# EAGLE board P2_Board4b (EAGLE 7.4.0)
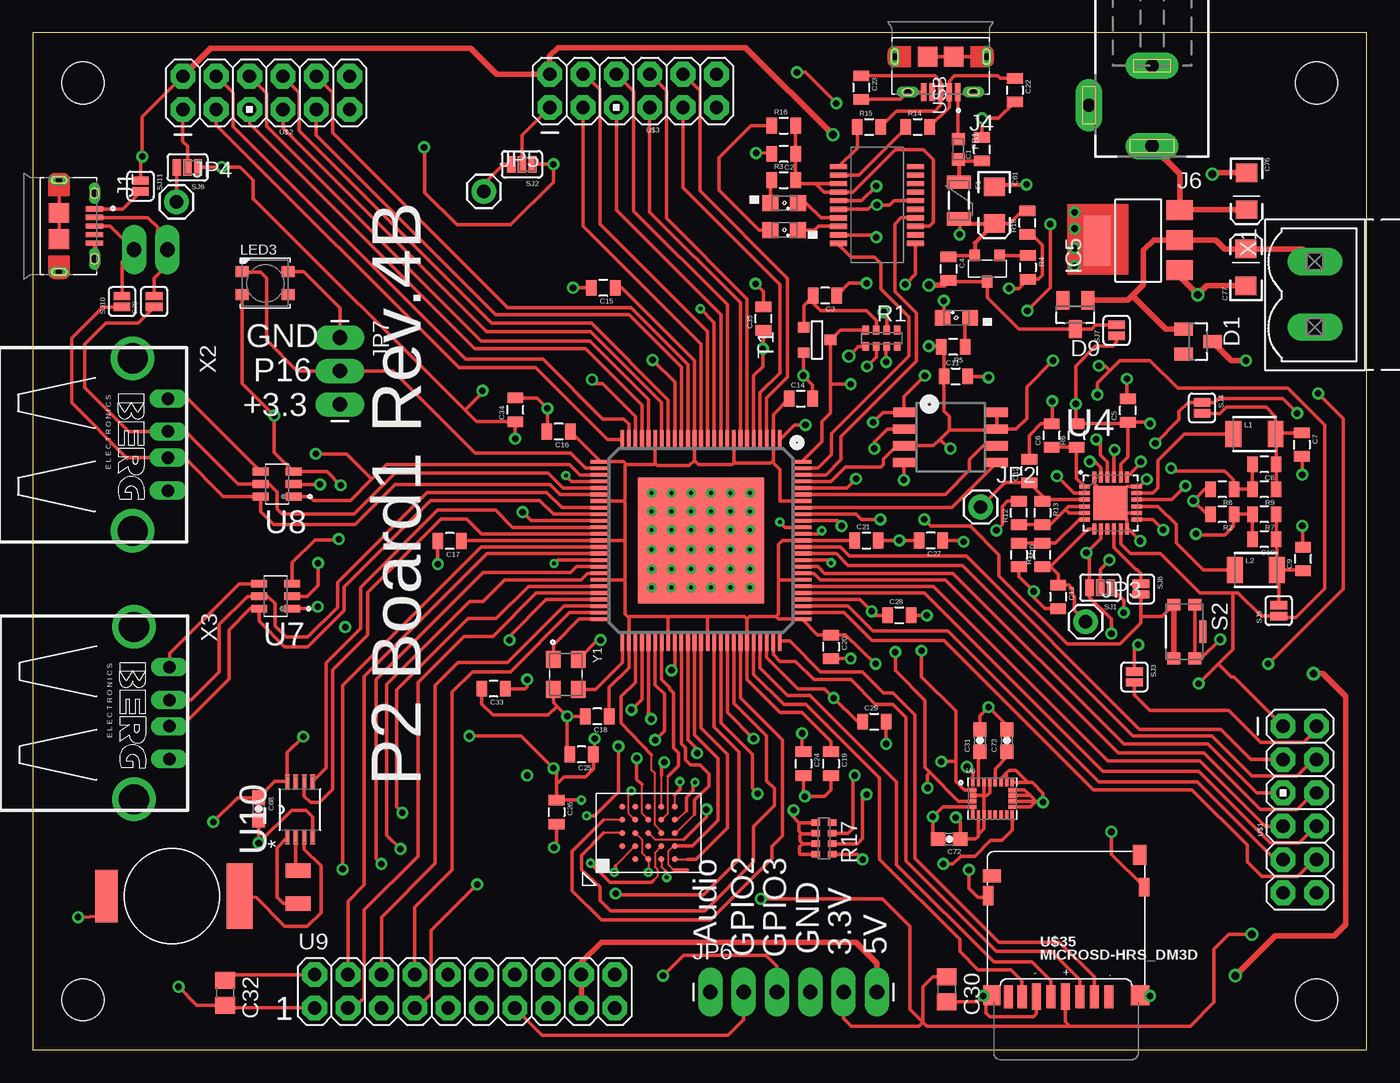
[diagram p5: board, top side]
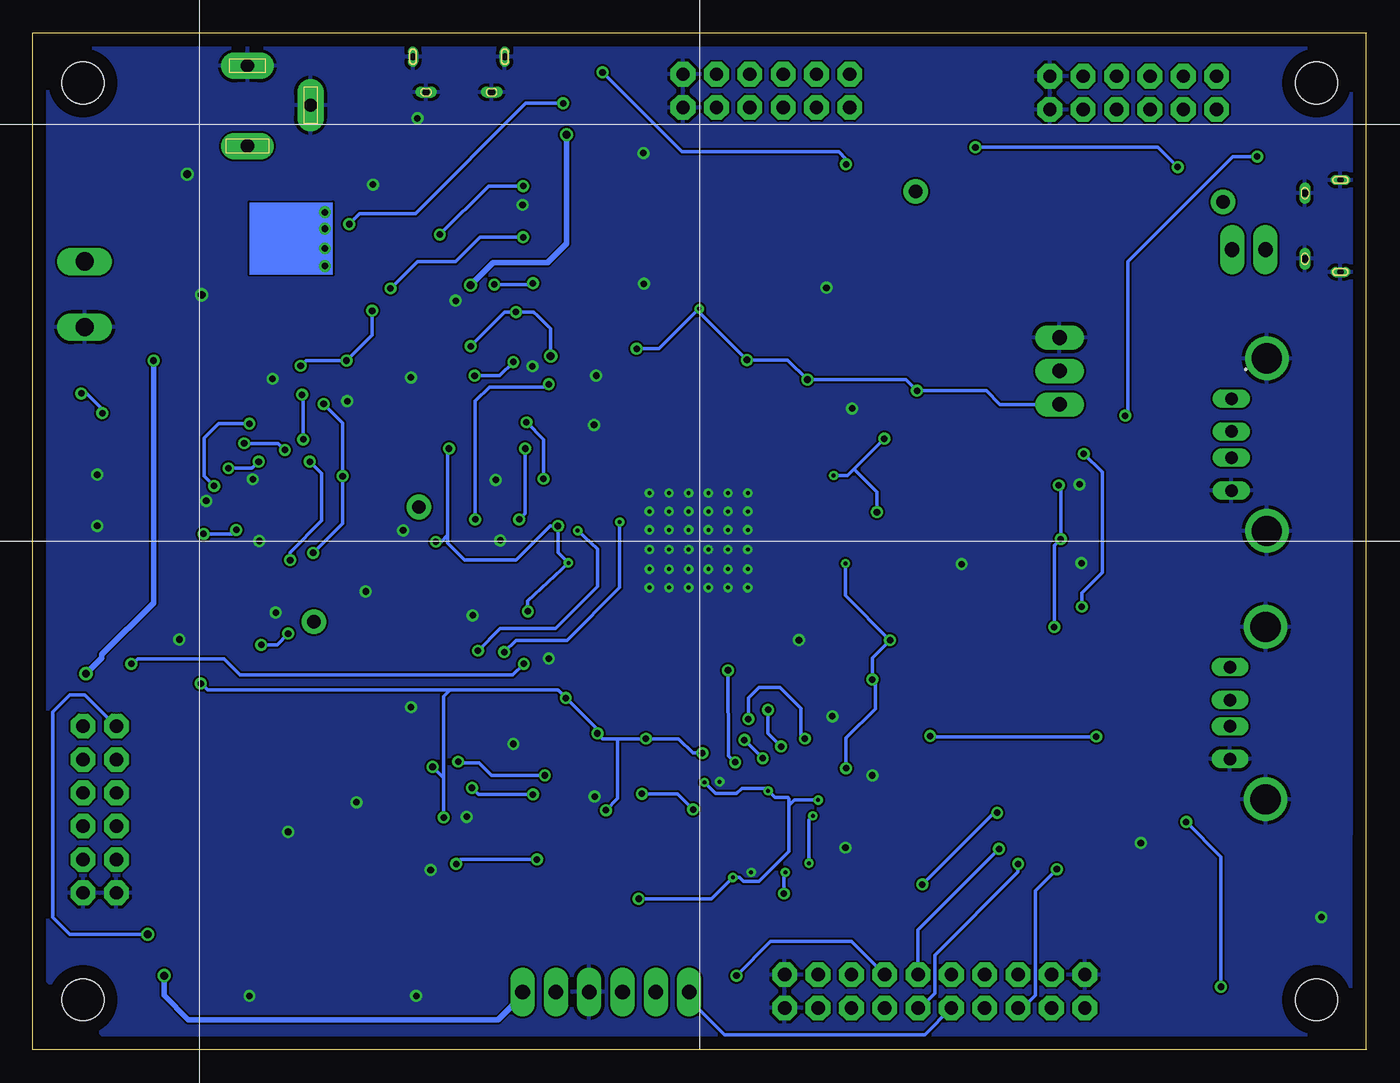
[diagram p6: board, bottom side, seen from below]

Size 101.6 x 77.47 mm. Coordinates in mm from the lower left corner, seen from the top.
Outline: 0.05,77.47 101.6,77.47 101.6,0 0.05,0
Outline: 0.05,77.47 0,77.47
Outline: 0,0 0.05,0
Outline: 0.05,0 0.05,77.47
Copper layers (1*16): Top 0.035mm / dielectric 1.5mm / Bottom 0.035mm
Design rules "default *": minimum track width 5mil, minimum drill 8mil, track to track 6mil, track to pad 6mil, pad to pad 6mil, via to via 8mil, smd to smd 8mil, copper to edge 40mil, drill to drill 8mil, minimum pad ring 4mil, minimum via ring 8mil, stop-mask expansion 4mil, vias tented up to drill 0mil, thermal gap 10mil
Net classes: 1 power: width 0.254 mm
Holes 3.2 mm at 3.81,3.81 3.81,73.66 97.79,73.66 97.79,3.81

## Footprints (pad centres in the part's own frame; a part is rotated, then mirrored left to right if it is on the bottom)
0805 = smd 0.8 x 1.2: 1 -0.9,0; 2 0.9,0
C0805 = smd 1.3 x 1.5: 1 -0.95,0; 2 0.95,0
0603-CAP = smd 1.1 x 1: 1 -0.85,0; 2 0.85,0
EIA3216 = smd 1.4 x 1.6: A 1.4,0; C -1.4,0
RAY2_SUPERCAP = smd 4 x 1.7: PNEG 0,0 | smd 5 x 2: PPOS 0,10.15
SOT23 = smd 1 x 1.4: 1 -0.95,-1.1; 2 0.95,-1.1; 3 0,1.1
PTC-1206 = smd 1 x 1.8: 1 -1.4,0; 2 1.4,0
INDC1608X80 = smd 0.92 x 0.98: 1 -0.775,0; 2 0.775,0
SOT223 = smd 1.499 x 2.007: 1 -2.261,-3.15; 2 0.025,-3.15; 3 2.311,-3.15 | smd 3.81 x 2.007: 4 0,3.15
AMPHENOL_10118194-0001LF = smd 0.4 x 1.35: 1 -1.3,2.7; 2 -0.65,2.7; 3 0,2.7; 4 0.65,2.7; 5 1.3,2.7 | drill 0.55 pad 0.65 long: S1 -2.5,2.7; S2 2.5,2.7 | drill 0.5 pad 0.775 long: S3 -3.5,0; S6 3.5,0 | smd 1.5 x 1.55: S4 -1,0; S5 1,0
DCJ0202 = drill 1 pad 2 long: 1 0,3.1; 2 4.8,0; 3 0,-3
1X01 = drill 1.016 pad 1.88: 1 0,0
1X06_LONGPADS = drill 1.118 pad 1.88 long: 1 0,0; 2 2.54,0; 3 5.08,0; 4 7.62,0; 5 10.16,0; 6 12.7,0
1X03_LONGPADS = drill 1.118 pad 1.88 long: 1 0,0; 2 2.54,0; 3 5.08,0
1X02_LONGPADS = drill 1.118 pad 1.88 long: 1 0,0; 2 2.54,0
1210 = smd 1.2 x 2: 1 -1.6,0; 2 1.6,0
SML0805 = smd 1.2 x 1.2: A 1.05,0; C -1.05,0
LED3535 = smd 1 x 0.85: 1 -1.75,0.875; 2 -1.75,-0.875; 3 1.75,-0.875; 4 1.75,0.875
MICRO3 = smd 0.8 x 0.9: 1 -0.95,-1; 2 0.95,-1; 3 0,1
0603-ARV = smd 0.5 x 0.65: 1 -1.2,-0.625; 2 -0.4,-0.625; 3 0.4,-0.625; 4 1.2,-0.625; 5 1.2,0.625; 6 0.4,0.625; 7 -0.4,0.625; 8 -1.2,0.625
SW_KMR221GLFS = smd 0.9 x 1: 1 -2.05,0.8; 2 -2.05,-0.8; 3 2.05,-0.8; 4 2.05,0.8 | smd 1.7 x 0.55: 5 0,1.425
SJ_3_PASTE1&2 = smd 0.635 x 1.27: 1 -0.813,0; 2 0,0; 3 0.813,0
SJ_2S = smd 0.635 x 1.27: 1 -0.412,0; 2 0.412,0
SOT-23 = smd 0.787 x 0.889: 1 0.025,-1.016; 2 -0.94,1.016; 3 0.991,1.016
SSOP20 = smd 0.4 x 1.3: 1 -2.925,-2.925; 2 -2.275,-2.925; 3 -1.625,-2.925; 4 -0.975,-2.925; 5 -0.325,-2.925; 6 0.325,-2.925; 7 0.975,-2.925; 8 1.625,-2.925; 9 2.275,-2.925; 10 2.925,-2.925; 11 2.925,2.925; 12 2.275,2.925; 13 1.625,2.925; 14 0.975,2.925; 15 0.325,2.925; 16 -0.325,2.925; 17 -0.975,2.925; 18 -1.625,2.925; 19 -2.275,2.925; 20 -2.925,2.925
PROPELLER_2 = smd 1.49 x 0.28: 1 -7.67,6; 2 -7.67,5.5; 3 -7.67,5; 4 -7.67,4.5; 5 -7.67,4; 6 -7.67,3.5; 7 -7.67,3; 8 -7.67,2.5; 9 -7.67,2; 10 -7.67,1.5; 11 -7.67,1; 12 -7.67,0.5; 13 -7.67,0; 14 -7.67,-0.5; 15 -7.67,-1; 16 -7.67,-1.5; 17 -7.67,-2; 18 -7.67,-2.5; 19 -7.67,-3; 20 -7.67,-3.5; 21 -7.67,-4; 22 -7.67,-4.5; 23 -7.67,-5; 24 -7.67,-5.5; 25 -7.67,-6; 51 7.67,-6; 52 7.67,-5.5; 53 7.67,-5; 54 7.67,-4.5; 55 7.67,-4; 56 7.67,-3.5; 57 7.67,-3; 58 7.67,-2.5; 59 7.67,-2; 60 7.67,-1.5; 61 7.67,-1; 62 7.67,-0.5; 63 7.67,0; 64 7.67,0.5; 65 7.67,1; 66 7.67,1.5; 67 7.67,2; 68 7.67,2.5; 69 7.67,3; 70 7.67,3.5; 71 7.67,4; 72 7.67,4.5; 73 7.67,5; 74 7.67,5.5; 75 7.67,6 | smd 0.28 x 1.49: 26 -6,-7.67; 27 -5.5,-7.67; 28 -5,-7.67; 29 -4.5,-7.67; 30 -4,-7.67; 31 -3.5,-7.67; 32 -3,-7.67; 33 -2.5,-7.67; 34 -2,-7.67; 35 -1.5,-7.67; 36 -1,-7.67; 37 -0.5,-7.67; 38 0,-7.67; 39 0.5,-7.67; 40 1,-7.67; 41 1.5,-7.67; 42 2,-7.67; 43 2.5,-7.67; 44 3,-7.67; 45 3.5,-7.67; 46 4,-7.67; 47 4.5,-7.67; 48 5,-7.67; 49 5.5,-7.67; 50 6,-7.67; 76 6,7.67; 77 5.5,7.67; 78 5,7.67; 79 4.5,7.67; 80 4,7.67; 81 3.5,7.67; 82 3,7.67; 83 2.5,7.67; 84 2,7.67; 85 1.5,7.67; 86 1,7.67; 87 0.5,7.67; 88 0,7.67; 89 -0.5,7.67; 90 -1,7.67; 91 -1.5,7.67; 92 -2,7.67; 93 -2.5,7.67; 94 -3,7.67; 95 -3.5,7.67; 96 -4,7.67; 97 -4.5,7.67; 98 -5,7.67; 99 -5.5,7.67; 100 -6,7.67 | smd 9.6 x 9.6: EP 0,0
SOIC_8_WIDE = smd 0.7 x 1.65: 1 -1.905,-3.533; 2 -0.635,-3.545; 3 0.635,-3.545; 4 1.905,-3.545; 5 1.905,3.545; 6 0.635,3.545; 7 -0.635,3.545; 8 -1.905,3.545
QFN50P400X400X100-25N = smd 0.813 x 0.305: 1 -1.981,1.245; 2 -1.981,0.762; 3 -1.981,0.254; 4 -1.981,-0.254; 5 -1.981,-0.762; 6 -1.981,-1.245; 13 1.981,-1.245; 14 1.981,-0.762; 15 1.981,-0.254; 16 1.981,0.254; 17 1.981,0.762; 18 1.981,1.245 | smd 0.305 x 0.813: 7 -1.245,-1.981; 8 -0.762,-1.981; 9 -0.254,-1.981; 10 0.254,-1.981; 11 0.762,-1.981; 12 1.245,-1.981; 19 1.245,1.981; 20 0.762,1.981; 21 0.254,1.981; 22 -0.254,1.981; 23 -0.762,1.981; 24 -1.245,1.981 | smd 2.591 x 2.591: 25 -0.025,0
TFBGA24 = smd 0.45 x 0.45: P$2 1,0; P$3 2,0; P$4 3,0; P$5 4,0; P$6 0,-1; P$7 1,-1; P$8 2,-1; P$9 3,-1; P$10 4,-1; P$11 0,-2; P$12 1,-2; P$13 2,-2; P$14 3,-2; P$15 4,-2; P$16 0,-3; P$17 1,-3; P$18 2,-3; P$19 3,-3; P$20 4,-3; P$21 0,-4; P$22 1,-4; P$23 2,-4; P$24 3,-4; P$25 4,-4
PQFN43P300X350X102-24N = smd 0.28 x 0.53: 1 -1.505,1.22; 6 -1.505,-1.22; 7 -1.075,-1.22; 8 -0.645,-1.22; 9 -0.215,-1.22; 10 0.215,-1.22; 11 0.645,-1.22; 12 1.075,-1.22; 13 1.505,-1.22; 18 1.505,1.22; 19 1.075,1.22; 20 0.645,1.22; 21 0.215,1.22; 22 -0.215,1.22; 23 -0.645,1.22; 24 -1.075,1.22 | smd 0.53 x 0.28: 2 -1.47,0.645; 3 -1.47,0.215; 4 -1.47,-0.215; 5 -1.47,-0.645; 14 1.47,-0.645; 15 1.47,-0.215; 16 1.47,0.215; 17 1.47,0.645
SOT95P280X145-6N = smd 1.21 x 0.58: 1 -1.255,0.95; 2 -1.255,0; 3 -1.255,-0.95; 4 1.255,-0.95; 5 1.255,0; 6 1.255,0.95
2X10 = drill 1.016 pad 1.88 octagon: 1 -11.43,-1.27; 2 -11.43,1.27; 3 -8.89,-1.27; 4 -8.89,1.27; 5 -6.35,-1.27; 6 -6.35,1.27; 7 -3.81,-1.27; 8 -3.81,1.27; 9 -1.27,-1.27; 10 -1.27,1.27; 11 1.27,-1.27; 12 1.27,1.27; 13 3.81,-1.27; 14 3.81,1.27; 15 6.35,-1.27; 16 6.35,1.27; 17 8.89,-1.27; 18 8.89,1.27; 19 11.43,-1.27; 20 11.43,1.27
SOP65P490X110-8N = smd 1.067 x 0.356: 1 -2.134,0.965; 2 -2.134,0.33; 3 -2.134,-0.33; 4 -2.134,-0.965; 5 2.134,-0.965; 6 2.134,-0.33; 7 2.134,0.33; 8 2.134,0.965
6X2HEADER = drill 1.016 pad 1.88 octagon: 1 -1.27,6.35; 2 1.27,6.35; 3 -1.27,3.81; 4 1.27,3.81; 5 -1.27,1.27; 6 1.27,1.27; 7 -1.27,-1.27; 8 1.27,-1.27; 9 -1.27,-3.81; 10 1.27,-3.81; 11 -1.27,-6.35; 12 1.27,-6.35
DM3D = smd 0.7 x 1.75: CD/DAT3 8.15,0.45; CLK 4.85,0.45; CMD 7.05,0.45; DAT0 2.65,0.45; DAT1 1.6,0.45; DAT2 9.25,0.45 | smd 0.8 x 1.5: GND1 0.05,8.15 | smd 0.8 x 1.4: GND2 11.95,8.8 | smd 1.4 x 1.5: GND3 11.65,0.55 | smd 1.3 x 1.5: GND4 0.35,0.55 | smd 1 x 1.55: SW_A 11.6,11.25 | smd 1.4 x 1: SW_B 0.35,9.65 | smd 0.7 x 2.032: VDD 5.95,0.45; VSS 3.75,0.45
MSTBV2 = drill 1.397 long: 1 -2.5,0; 2 2.5,0
PN87520-S = drill 0.95 long: 1 -3.5,2.71; 2 -1,2.71; 3 1,2.71; 4 3.5,2.71 | drill 2.3 pad 2.9: S1 -6.57,0; S2 6.57,0
RAY2_SMT_CRYSTAL = smd 1.1 x 1.9: P$1 0,0; P$2 2.5,0
XTAL_ECS-200-9-33B-CKY-TR = smd 1.3 x 1.1: 1 -1.15,-0.95; 2 1.15,-0.95; 3 1.15,0.95; 4 -1.15,0.95

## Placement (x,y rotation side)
C1  0.1uF  [0805]  72.3,68.6 90 top
C2  0.1uF  [0805]  57.2,68.25 180 top
C3  0.1uF  [0805]  60.35,57.45 180 top
C4  0.1uF  [0805]  69.75,59.5 270 top
C5  10uF  [0805]  83.4,48.7 90 top
C6  0.1uF  [0805]  77.6,46.8 90 top
C7  10uF  [0805]  96.65,46.1 270 top
C8  47p  [0805]  93.8,44.6 180 top
C9  10uF  [0805]  96.75,37.4 90 top
C10  47p  [0805]  93.8,38.9 180 top
C11  0.1uF  [0805]  70.3,51.3 0 top
C12  10uF  [0805]  75.9,44.1 90 top
C13  10uF  [0805]  78.1,34.5 270 top
C14  1uF  [0805]  58.5,49.6 0 top
C15  1uF  [0805]  43.45,58.05 180 top
C16  1uF  [0805]  40.05,47.1 180 top
C17  1uF  [0805]  31.75,38.75 180 top
C18  1uF  [0805]  43,25.4 180 top
C19  1uF  [0805]  60.8,21.8 270 top
C20  1uF  [0805]  60.8,30.7 270 top
C21  1uF  [0805]  63.5,38.8 0 top
C22  47p  [0805]  74.8,73.1 270 top
C23  47p  [0805]  63.1,73.3 270 top
C24  1uF  [0805]  58.7,21.8 270 top
C25  1uF  [0805]  41.8,22.5 180 top
C26  1uF  [0805]  39.9,18.1 270 top
C27  1uF  [0805]  68.4,38.8 180 top
C28  1uF  [0805]  66,33.1 0 top
C29  1uF  [0805]  64.1,25 0 top
C30  1u  [C0805]  69.6,4.6 270 top
C31  0.1u  [0603-CAP]  72.15,23.55 90 top
C32  1u  [C0805]  14.65,4.35 270 top
C33  1uF  [0805]  35.1,27.5 180 top
C34  1uF  [0805]  36.75,48.75 90 top
C35  1uF  [0805]  55.65,55.7 90 top
C61  10uF  [EIA3216]  73.24,64.34 270 top
C68  1u  [0603-CAP]  17.2,18.35 270 top
C71  RAY2_SUPERCAP  [RAY2_SUPERCAP]  5.6,11.7 270 top
C72  1uF  [0603-CAP]  69.8,16.05 180 top
C73  0.1u  [0603-CAP]  74.2,23.55 90 top
C76  10uF  [EIA3216]  92.45,65.4 270 top
C77  10uF  [EIA3216]  92.4,59.6 90 top
D1  BAS40  [SOT23]  88.75,53.95 270 top
D9  BAS40  [SOT23]  79.4,56 180 top
F1  500mA  [PTC-1206]  70.54,64.69 270 top
FB1  MPZ1608S221ATA00  [INDC1608X80]  70.5,68.6 270 top
IC5  REG1117  [SOT223]  84.2,61.65 90 top
J1  10118194-0001LF  [AMPHENOL_10118194-0001LF]  2,62.75 270 top
J4  10118194-0001LF  [AMPHENOL_10118194-0001LF]  69.15,75.65 180 top
J6  DCJ0202  [DCJ0202]  85.25,71.95 180 top
JP2  M01PTH  [1X01]  72.2,41.35 0 top
JP3  M01PTH  [1X01]  80.2,32.6 0 top
JP4  M01PTH  [1X01]  10.95,64.6 0 top
JP5  M01PTH  [1X01]  34.35,65.4 0 top
JP6  [1X06_LONGPADS]  51.6,4.4 0 top
JP7  [1X03_LONGPADS]  23.4,54.25 270 top
JP8  M02PTH3  [1X02_LONGPADS]  10.25,60.95 180 top
L1  3.3uH  [1210]  93.05,46.9 0 top
L2  3.3uH  [1210]  93.15,36.55 0 top
LED1  Red  [SML0805]  57.24,62.45 180 top
LED2  Green  [SML0805]  57.24,64.5 180 top
LED3  WS2812B3535  [LED3535]  17.7,58.4 0 top
LED5  Yellow  [SML0805]  70.34,55.76 0 top
Q3  IRLML5203  [MICRO3]  72.69,59.51 180 top
R1  10k  [0603-ARV]  64.65,54.2 180 top
R2  150k  [0805]  90.6,40.8 180 top
R3  100  [0805]  57.2,66.25 0 top
R4  1k  [0805]  75.8,59.6 270 top
R5  100  [0805]  70.1,53.55 180 top
R6  1  [0805]  79.5,46.8 90 top
R7  680k  [0805]  93.8,40.8 180 top
R8  150k  [0805]  90.6,42.7 180 top
R9  300k  [0805]  93.8,42.7 180 top
R10  130k  [0805]  75.1,37.7 270 top
R11  300k  [0805]  76.9,37.7 90 top
R12  130k  [0805]  75.1,40.9 90 top
R13  300k  [0805]  76.9,40.9 270 top
R14  27  [0805]  67.4,70.3 0 top
R15  27  [0805]  63.7,70.3 0 top
R16  100  [0805]  57.2,70.4 0 top
R17  10k  [0603-ARV]  60.25,16.1 90 top
R18  10k  [0805]  75.75,63 90 top
S2  KMR221GLFS  [SW_KMR221GLFS]  87.7,31.85 270 top
SJ1  [SJ_3_PASTE1&2]  81.3,35.2 180 top
SJ2  [SJ_3_PASTE1&2]  37.25,67.45 180 top
SJ3  SOLDERJUMPERNC  [SJ_2S]  83.9,28.4 270 top
SJ4  SOLDERJUMPERNC  [SJ_2S]  89.05,48.9 270 top
SJ5  SOLDERJUMPERNC  [SJ_2S]  94.9,33.45 90 top
SJ6  [SJ_3_PASTE1&2]  11.78,67.21 180 top
SJ7  SOLDERJUMPERNC  [SJ_2S]  82.55,54.8 90 top
SJ8  SOLDERJUMPERNC  [SJ_2S]  84.4,35.1 270 top
SJ9  SOLDERJUMPERNC  [SJ_2S]  9.25,57 90 top
SJ10  SOLDERJUMPERNC  [SJ_2S]  6.8,57 90 top
SJ11  SOLDERJUMPERNC  [SJ_2S]  8.2,65.8 270 top
T1  2N3904  [SOT-23]  59.74,54.05 90 top
U1  FT231XS-R  [SSOP20]  64.3,64.35 90 top
U2  Propeller 2 - ES  [PROPELLER_2]  50.9,38.8 270 top
U3  SPI Flash 16MB (128Mb)  [SOIC_8_WIDE]  69.9,46.65 270 top
U4  TPS650532RGER  [QFN50P400X400X100-25N]  82.1,41.65 0 top
U5  HYPERRAM  [TFBGA24]  44.89,14.52 90 top
U6  LSM9DS1TR  [PQFN43P300X350X102-24N]  73.1,19.15 0 top
U7  TPD3S014DBVR  [SOT95P280X145-6N]  18.5,34.55 180 top
U8  TPD3S014DBVR  [SOT95P280X145-6N]  18.6,43.1 180 top
U9  M10X2  [2X10]  32.9,4.45 0 top
U10  DS1342U+  [SOP65P490X110-8N]  20.35,18.3 90 top
U$1  2X6HEADER  [6X2HEADER]  96.5,18.3 0 top
U$2  2X6HEADER  [6X2HEADER]  17.78,72.9 90 top
U$3  2X6HEADER  [6X2HEADER]  45.72,73.05 90 top
U$35  MICROSD-HRS_DM3D  [DM3D]  72.7,3.6 0 top
X1  [MSTBV2]  97.65,57.55 270 top
X2  PN87520-S  [PN87520-S]  7.6,46.1 270 top
X3  PN87520-S  [PN87520-S]  7.7,25.65 270 top
X5  RAY2_SMT_CRYSTAL  [RAY2_SMT_CRYSTAL]  20.2,13.65 270 top
Y1  ECS-200-9-33B-CKY-TR  [XTAL_ECS-200-9-33B-CKY-TR]  40.6,28.6 270 top

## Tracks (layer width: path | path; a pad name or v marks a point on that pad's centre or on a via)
1.8V  (via drill 0.5)
  Top 0.254: U4.21 82.35,45.65 v82.4,45.7 | U2.94 56.9,41.8 56.9,44.2 56.4,44.7 56.4,44.9 | 56.4,44.9 U2.2 56.4,48.4 C14.1 | U2.8 53.4,44.7 | 53.4,44.7 56.2,44.7 56.4,44.9 | 50.4,44.9 U2.14 50.4,52.5 44.85,58.05 C15.1 | 50.4,44.9 50.7,44.6 53.3,44.6 53.4,44.7 | U2.20 47.4,44.7 | 47.4,44.7 47.6,44.5 50,44.5 50.4,44.9 | 45.2,44.6 45,44.8 U2.26 43.23,44.82 C16.1 | 45.2,44.6 47.3,44.6 47.4,44.7 | U2.32 45,41.8 | 45,41.8 45.1,41.9 45.1,44.5 45.2,44.6 | 45.1,38.8 U2.38 33.2,38.8 C17.1 | 45.1,38.8 45.1,41.7 45,41.8 | U2.44 45,35.8 | 45,35.8 45.1,35.9 45.1,38.8 | 45.4,32.9 U2.52 45.4,29.1 43.9,27.6 C18.1 | 45.4,32.9 45.1,33.2 45.1,35.7 45,35.8 | U2.58 48.4,32.9 | 48.4,32.9 48.3,33 45.5,33 45.4,32.9 | U2.64 51.4,33 | 51.4,33 48.5,33 48.4,32.9 | 54.4,32.8 U2.70 54.4,28.2 56.9,25.7 58.6,25.7 60.8,23.5 C19.1 | 54.4,32.8 54.2,33 51.4,33 | 56.6,33 56.8,32.8 U2.76 59.77,31.6 C20.1 61.9,31.6 v64.2,29.4 | 56.6,33 54.6,33 54.4,32.8 | U2.82 56.9,35.8 | 56.9,35.8 56.8,35.7 56.8,33.2 56.6,33 | 56.9,35.8 56.8,35.9 56.8,38.5 57.1,38.8 U2.88 C21.1 | v94.1,29.4 99.8,35.1 99.8,48.1 v97.9,50 | v85.5,46.2 87.3,48 87.3,48.6 88.01,49.31 SJ4.1 90.01,49.31 90.3,49.6 95.2,49.6 v96.3,48.5
  Bottom 0.254: v82.4,45.7 82.9,46.2 v85.5,46.2 | v97.9,50 97.5,50 96,48.5 v96.3,48.5 | v64.2,29.4 65.05,28.55 85.8,28.55 87.03,29.77 93.62,29.77 94,29.4 v94.1,29.4
3V3OUT
  Top 0.254: 58.33,65.97 R3.2 | U1.13 59.6,65.97 | 59.6,65.97 58.38,65.97 R3.2 | R3.2 C2.1 R16.2 | 59.6,65.97 60.25,65.33 U1.14 62.48,65.33 65.7,68.55 67.85,68.55 68.6,67.8 68.6,63.05 68.28,62.73 U1.3
5V_USB  (via drill 0.5)
  Top 0.254: Q3.2 69.91,60.51 C4.1 | U1.15 63.12,64.67 v64.25,65.8 | F1.2 70.6,63.23 v70.6,62.1 | C61.A 74.39,62.95 75.35,63.9 R18.2
  Top 0.305: F1.2 70.94,62.9 72.6,62.9 72.64,62.95 C61.A 71.75,61.45 Q3.2
  Bottom 0.254: v70.6,62.1 66.9,65.8 v64.25,65.8
+3V3  (via drill 0.3, 0.3 pad 0.3, 0.5, 0.5 pad 0.3, 0.51 pad 0.3, 0.6)
  Top 0.152: U5.P$24 49.09,17.52 49.79,18.22 | U5.P$9 45.39,18.02 45.39,19.52 | U5.P$16 47.89,13.92 48.19,13.62
  Top 0.254: U4.11 82.86,38.54 83.6,37.8 85.9,37.8 88.9,34.8 91.4,34.8 | U4.22 81.85,44.75 81.3,45.3 81.3,46.2 v81,46.5 | v81.1,49.9 81.1,50.8 82.05,51.75 | 82.05,51.75 82.8,52.5 85.1,52.5 87.2,50.4 95.6,50.4 98.4,47.6 98.4,35.15 96.2,32.95 94.99,32.95 SJ5.1 93.56,33.04 91.8,34.8 91.4,34.8 | U3.7 74.89,47.28 75.7,48.1 75.7,50.5 v77.7,52.5 | v81.2,52.1 81.7,52.1 82.05,51.75 | 69.8,47.2 69.1,46.5 | 69.1,46.5 68.61,46.02 U3.3 65.81,46.02 64.8,45 64.8,44.6 64.6,44.4 61.9,44.4 60.8,43.3 U2.97 | U3.8 U3.7 | 49.79,18.22 49.79,19.22 50.29,19.72 50.29,20.22 v50.44,20.37 50.49,20.42 | 45.39,19.52 v45.59,19.72 | 48.19,13.62 48.19,13.22 v48.29,13.12 | U2.55 46.9,25.4 v47.1,25.2 | v42.8,23.7 42.8,22.6 C25.1 42.7,21.4 42.1,20.8 40.47,20.8 39.9,20.23 | U2.61 49.9,23.6 50.7,22.8 50.7,22.7 v50.6,22.6 | U2.67 52.9,25.7 v54.9,23.7 | v58.6,24.1 58.6,22.8 C24.1 | v41.79,19.02 39.92,19.02 C26.1 39.9,20.23 | U2.91 61.3,40.3 v61.6,39.9 | v69.9,45.8 69.8,45.8 69.1,46.5 | C27.1 70.8,38.8 v70.9,38.7 | U2.79 63,34.3 v63.9,33.4 64.2,33.1 C28.1 | v60.8,37.1 60.6,37.3 U2.85 | U2.73 55.9,29.9 58.3,27.5 60.3,27.5 v61,26.8 62.8,25 C29.1 | v88.8,27.9 90.25,29.35 | 90.25,29.35 91.4,30.5 91.4,34.8 | 79,1.8 68.1,1.8 67.8,2.1 | 79,1.8 88.15,1.8 89.95,3.6 89.95,7.65 91.1,8.8 v92.85,8.8 | 90.25,29.35 90.35,29.35 91.3,28.4 91.48,28.4 U$1.1 | U$35.VDD 78.65,2.15 79,1.8 | C30.1 68.55,5.55 67.8,4.8 67.8,2.1 | 72.03,16.4 72.03,16.27 71.8,16.05 C72.1 70.65,17.35 v70.3,17.7 | 72.03,16.4 U6.7 | 72.03,16.4 72.45,16.83 U6.8 72.45,19.32 72.5,19.36 | U6.22 72.89,19.59 72.67,19.36 72.6,19.36 | 72.6,19.36 72.5,19.36 | 72.5,19.36 U6.3 | U6.23 72.45,19.51 72.6,19.36
  Top 0.254: U6.1 71.59,21.11 v71.15,21.55 | R17.5 58.35,17.3 | 58.35,17.3 57.85,17.8 57.85,18.15 v57.95,18.25 | R17.6 59.58,16.45 58.55,16.45 | 58.55,16.45 58.35,16.65 58.35,17.3 | R17.7 58.65,15.7 | 58.65,15.7 58.45,15.9 58.45,16.35 58.55,16.45 | R17.8 58.45,14.9 58.4,14.95 58.4,15.45 58.65,15.7 | 67.8,2.1 66.8,3.1 66.8,9.4 64.7,11.5 62.3,11.5 | 62.3,11.5 v55.45,11.5 | v36.3,31.2 36.3,31.5 39.1,34.3 U2.47 | U2.41 39.95,37.3 v39.7,37.05 | v58.2,74.45 58.85,74.45 v61.2,72.1 | v77.5,62.9 77.5,58.05 v75.75,56.3 | 16.8,64.8 16.8,64.85 | 16.8,64.85 16.8,66.26 15.81,67.25 v14.4,67.25 12.63,67.25 SJ6.1 | 32.92,48.73 33.8,47.85 C34.1 v36.75,46.55 | U2.29 41.05,43.3 v40.6,43.75 | U2.35 37.95,40.3 v37.3,40.95 | U2.23 45.9,48.25 43.4,50.75 42.9,50.75 v42.6,51.05 | v34.25,50.2 34.25,50.05 32.92,48.73 | U2.17 48.9,50.85 v47.2,52.55 | U2.11 51.9,55.4 v50.85,56.45 | U2.5 54.9,51.35 55.6,52.05 v55.6,53.4 55.65,53.45 C35.1 | SJ2.1 v39.65,67.45 39.65,66.1 36.4,62.85 32.3,62.85 29.85,65.3 29.85,68.7 v29.8,68.75 | U3.7 73.36,47.2 69.8,47.2 | 69.8,47.2 69.8,48.25 69.4,48.65 C11.1 69.4,53.35 R5.2 | R1.5 62.88,53.58 v62.15,52.85 | 32.92,48.73 16.8,64.85 | 36,27.4 C33.1 37.5,27.5 37.65,27.65 v37.65,28.2 | 39.9,20.23 39.9,21.2 v39.65,21.45 37.2,23.9 v33.25,23.9 | v20.6,23.85 19.39,22.64 U10.8 18.43,20.43 C68.1 15.6,19.2 v13.75,17.35 | 62.26,11.46 62.3,11.5 | v11.1,4.8 12.5,3.4 C32.2 14.87,3.18 U9.1 | JP6.5 61.76,2.39 62.35,1.8 67.5,1.8 67.8,2.1 | v68.25,53.6 69.2,53.6 | R1.2 65.05,55.95 v64.8,56.2
  Top 0.406: 69.2,53.6 R5.2
  Bottom 0.254: v81,46.5 81,49.8 v81.1,49.9 | v81.2,52.1 80.8,52.5 v77.7,52.5 75.75,54.45 v75.75,56.3 | 43.99,18.62 43.99,15.12 46.29,12.82 47.49,12.82 47.79,13.12 v48.29,13.12 49.9,11.5 v55.45,11.5 | 43.99,18.62 43.99,19.12 44.09,19.22 45.09,19.22 v45.59,19.72 45.79,19.92 47.59,19.92 47.99,19.52 49.59,19.52 v50.44,20.37 | v41.79,19.02 43.59,19.02 43.99,18.62 | v47.1,25.2 47.1,26.8 46.3,27.6 44.7,27.6 43.1,26 43.1,24 v42.8,23.7 | v50.6,22.6 51.3,22.6 52.4,23.7 v54.9,23.7 57.05,23.7 | 57.05,23.7 58.2,23.7 v58.6,24.1 58.6,24.4 v61,26.8 61.6,27.4 69.8,27.4 | 70,39.2 70,38.6 68.7,37.3 64.8,37.3 62.2,39.9 v61.6,39.9 61.6,37.9 v60.8,37.1 63.9,34.2 v63.9,33.4 | 70,39.2 70,45.7 v69.9,45.8 | v70.9,38.7 70.5,38.7 70,39.2 | 69.8,27.4 88.3,27.4 v88.8,27.9 | v71.15,21.55 70.3,20.7 | 70.3,20.7 v70.3,17.7 | 70.3,20.7 70.3,26.9 69.8,27.4 | v57.95,18.25 57.05,19.15 57.05,23.7 | v39.7,37.05 39.7,34.6 v36.3,31.2 37.65,29.85 v37.65,28.2 37.42,27.98 37.42,25.98 39.65,23.75 v39.65,21.45 | v58.2,74.45 52.15,68.4 40.2,68.4 39.65,67.85 v39.65,67.45 | v61.2,72.1 64.05,72.1 72.45,63.7 76.7,63.7 v77.5,62.9 | v40.6,43.75 39.55,43.75 39.05,44.25 | 39.05,44.25 v36.75,46.55 | v37.3,40.95 37.3,42.5 39.05,44.25 | v55.6,53.4 53.9,53.4 v50.85,56.45 50.85,56.2 v47.2,52.55 44.1,52.55 v42.6,51.05 35.1,51.05 v34.25,50.2 28.95,50.2 27.92,49.17 JP7.3 | 14.55,67.4 v14.4,67.25 15.9,68.75 v29.8,68.75 | v20.6,23.85 33.2,23.85 v33.25,23.9 | v13.75,17.35 11.1,14.7 v11.1,4.8 | v68.25,53.6 65.65,56.2 v64.8,56.2 63.45,56.2 63.1,55.9 62.15,54.95 v62.15,52.85 | v92.85,8.8 98.8,8.8 100.1,10.1 100.1,25.75 98.8,27.05 97.63,27.05 U$1.1
+5_VIN
  Top 0.406: 83.75,57.45 84.6,58.3 84.6,60.9 85.38,61.67 IC5.2 90.12,61.67 90.8,61 C77.A 96.7,61 X1.1 | 83.75,57.45 83.4,57.1 D9.1 | D1.1 86.3,54.9 83.75,57.45
+5V  (via drill 0.5, 0.51 pad 0.3, 0.6 pad 0.3)
  Top 0.254: C4.2 69.89,58.51 Q3.3 72.69,57.3 75.1,54.9 D9.3 | U$2.2 8.35,71.09 v8.35,68.05 8.2,67.9 SJ11.1 | U7.3 19.75,37.1 21.5,38.85 23.25,38.85 v23.3,38.9 | v23.45,43 22.4,44.05 U8.3 18.4,45.51 v18.4,48.3 15.95,50.75 LED3.2 | D9.3 79.3,54.8 | D9.3 80.65,54.9 80.95,55.2 82.54,55.2 SJ7.2
  Top 0.406: v60.95,69.7 54.3,76.35 40,76.35 39.37,75.72 U$3.2 35.33,74.32 33.35,76.3 13.56,76.3 U$2.2 | v68.25,58.25 69.4,58.25 C4.2
  Bottom 0.254: v8.35,68.05 10.2,68.05 18.2,60.05 18.2,48.5 v18.4,48.3 | v23.45,43 23.3,42.85 v23.3,38.9 23.8,38.4 v23.8,32.2
  Bottom 0.406: v60.95,69.7 60.95,61.4 62.4,59.95 66.55,59.95 v68.25,58.25
+5VPI  (via drill 0.5 pad 0.3, 0.6)
  Top 0.406: D1.3 91.3,52.5 v92.4,52.5 | U9.17 U9.18 41.79,6.69 43.3,8.2 62.7,8.2 64.3,6.6 JP6.6 | v91.6,5.65 94.65,8.7 99.15,8.7 100,9.55 100,26.9 98.25,28.65 v97.55,28.65
  Bottom 0.406: v92.4,52.5 92.4,34.05 96.35,30.1 96.35,29.85 v97.55,28.65 | JP6.6 64.3,4.15 66.15,2.3 89.75,2.3 91.6,4.15 v91.6,5.65
AUDIO1
  Bottom 0.254: JP6.1 51.6,3.85 48.9,1.15 33.66,1.15 U9.9
CSN
  Top 0.254: U2.48 40.45,33.8 36.15,29.5 32.4,29.5 30.65,27.75 30.65,14.2 26.55,10.1 U9.6
D1_N
  Top 0.254: U2.30 40.4,42.8 39.25,43.95 27.61,43.95 24.46,40.8 19,40.8 18.6,41.2 18.6,42.5 18,43.1 U8.5 15.65,43.1 11.65,47.1 X2.2 7.3,47.1 3.95,50.45 3.95,53.75 5.55,55.35 8.01,55.35 SJ9.1
D1_P
  Top 0.254: U2.31 40.15,42.3 39.4,43.05 27.59,43.05 24.54,40 18.35,40 17.34,41.01 U8.6 14.5,42.15 11.55,45.1 X2.3 7.25,45.1 7.2,45.05 2.95,49.3 2.95,54.2 5.34,56.59 SJ10.1
D2_N
  Top 0.254: X3.2 12.05,26.65 14.2,28.8 14.2,32.4 16.35,34.55 U7.5 17.9,34.55 18.45,34 18.45,32.3 19.3,31.45 20.95,31.45 23.2,33.7 23.2,35.6 30.05,42.45 39.15,42.45 40.3,41.3 U2.33
D2_P
  Top 0.254: U2.34 39.65,40.8 38.6,41.85 30.3,41.85 23.7,35.25 23.7,33.45 20.95,30.7 19.2,30.7 17.25,32.66 U7.6 16.55,33.6 14.95,32 14.95,28.25 11.35,24.65 X3.3
DTR  (via drill 0.5)
  Top 0.254: U1.1 67.22,59.08 v66.45,58.3 | v63.5,58.4 62.15,58.4 C3.1
  Bottom 0.254: v66.45,58.3 63.6,58.3 v63.5,58.4
FB_DCDC1  (via drill 0.5)
  Top 0.254: U4.19 84.4,44.69 v84.4,44.8 | v86.7,44.3 86.9,44.1 90.8,44.1 91.45,43.45 R8.1 R9.2 C8.2
  Bottom 0.254: v84.4,44.8 84.9,44.3 v86.7,44.3
FB_DCDC2  (via drill 0.5)
  Top 0.254: v88.6,39.3 88.7,39.2 90.8,39.2 91.45,39.85 R2.1 R7.2 C10.2 | v86.1,39.6 85.3,40.41 U4.13
  Bottom 0.254: v88.6,39.3 86.4,39.3 v86.1,39.6
FB_LDO1
  Top 0.254: U4.4 78.9,41.4 78.65,41.15 | 78.65,41.15 77.5,40 R13.2 R12.1 | U4.5 78.91,40.89 78.65,41.15
FB_LDO2
  Top 0.254: U4.6 79.7,40.41 77.9,38.6 R11.2 R10.1
FCLK
  Top 0.254: U3.6 72.42,46.02 71.35,44.95 71.35,44.15 69.5,42.3 U2.95
FCSN  (via drill 0.5)
  Top 0.254: U2.96 62,42.8 v62.7,43.5 | v64,47.8 64.75,48.55 U3.1 66.37,49.77 v67.95,51.35 | v65,52.4 65,53.52 R1.7
  Bottom 0.254: v62.7,43.5 62.7,46.5 v64,47.8 | v67.95,51.35 66.05,51.35 v65,52.4
FDI
  Top 0.254: U3.5 70,41.3 U2.93
FDO  (via drill 0.5)
  Top 0.254: U3.2 65.08,47.28 64.1,46.3 v64.1,45.8 | v64.55,40.4 63.1,40.4 62.7,40.8 U2.92
  Bottom 0.254: v64.1,45.8 64.1,40.85 v64.55,40.4
GND  (via drill 0.3, 0.3 pad 0.3, 0.3 pad 0.41, 0.5, 0.6)
  Top 0.152: 48.89,19.42 U5.P$25 | U5.P$8 46.39,16.02 46.39,15.02 U5.P$11 v46.89,13.52
  Top 0.254: U1.6 65.58,64.67 65.27,64.36 v64.3,64.36 63.97,64.36 63.63,64.03 U1.16 | 56.4,68.3 C2.2 56.4,68.34 v55.09,68.31 | T1.2 58.7,53.08 v58.7,51.36 59.4,50.66 C14.2 | R1.6 64.25,52.77 v63.55,52.06 | U3.4 66.34,44.73 v66.34,43.41 | C7.2 96.69,45.17 v96.69,43.81 | U4.18 83.32,42.9 U4.25 | U4.24 80.86,43.15 81.4,42.6 | 81.4,42.6 81.6,42.4 81.6,42.1 | v83.34,51.11 83.34,49.66 C5.2 | v96.69,39.91 96.75,39.85 C9.2 | C1.2 v72.3,70.95 v72.3,70.96 73.56,70.96 C22.2 | v77.64,49.41 77.64,47.74 C6.2 76.8,47.7 75.9,46.8 C12.2 | R2.2 89.41,40.8 v88.39,41.81 89.28,42.7 R8.2 | R10.2 75.1,36.05 v76.25,34.91 76.25,34.45 77.1,33.6 C13.2 | U4.14 82.84,40.89 U4.25 | U4.25 83.34,40.38 U4.12 83.44,39.67 v84.34,38.76 | Y1.4 43.01,31.21 v43.24,31.21 | C17.2 v30.85,37 | C18.2 v40.7,25.4 | C21.2 v66,38.8 C27.2 | C20.2 v62.3,29.8 | v41.15,58.05 C15.2 | C23.2 66.1,72.4 J4.S2 J4.5 | U2.EP 50.8,41.85 v50.15,42.41 | v49.29,20.42 49.29,19.82 48.89,19.42 | C25.2 40.7,22.7 v40.7,25.4 | C24.2 58.7,19.4 v58.8,19.3 60.3,19.3 60.8,19.8 C19.2 | C26.2 39.9,15.6 v39.7,15.4 | C28.2 v68.1,33.1 | C29.2 v65,23.3 | C30.2 71.95,3.65 v72.4,4.1 72.6,3.9 | U$35.VSS 76.45,2.75 76.2,2.5 72.9,2.5 72.6,2.8 72.6,3.9 | v71.3,13.7 71.3,12.3 72,11.6 72.6,11.6 U$35.GND1 | v85.1,4.1 84.4,4.1 U$35.GND3 | 72.6,3.9 72.6,4 72.4,4.2 73,4.2 U$35.GND4 | C31.2 72.15,25.45 v72.8,26.1 74.2,24.7 C73.2 | C72.2 68.55,16.45 v68.55,17.75 69.31,18.5 U6.5 71.59,18.5 U6.6 | U6.15 76.4,18.93 | 76.4,18.93 76.86,18.93 v76.95,18.85 76.95,19.55 76.13,20.37 75.8,20.37 | U6.14 75.97,18.5 76.4,18.93 | U6.16 75.97,19.36 | 75.97,19.36 76.4,18.93 | U6.17 75.54,19.8 75.97,19.36 | U6.18 75.8,20.37 | U6.19 74.17,21.07
  Top 0.254: 74.17,21.07 74.4,21.3 74.87,21.3 75.8,20.37 | U6.20 73.75,20.64 74.17,21.07 | Y1.2 39.65,26.45 39.92,26.18 | 39.92,26.18 v40.7,25.4 | C16.2 39.2,47.15 v39.2,48.85 38.4,49.65 C34.2 | U8.2 19.89,43.07 v21.87,43.07 | C35.2 55.65,57.75 v55.05,58.35 | v90.44,31.26 88.98,29.8 S2.4 S2.1 | U4.25 81.4,42.33 81.4,42.6 | C68.2 v17.2,15.75 19.7,18.25 20.8,18.25 21.32,17.73 U10.4 | v3.45,10.1 6.1,10.2 C71.PNEG | R12.2 74.25,41.8 73.85,41.4 73.85,40.02 v73.39,39.56 | 84.3,42.9 84.84,43.45 v84.84,43.46 | J4.S5 J4.S4 J4.S3 | C11.2 72.7,51.3 v72.8,51.21 | LED5.C 69.39,56.01 v69.39,57.06 | U2.1 58.03,47.6 v58.85,47.6 | SJ1.1 83.09,34.22 v83.09,33.31 | U$35.GND2 82.15,14.9 v82.15,16.6 | C33.2 34.2,26.35 35.05,25.5 39.25,25.5 39.92,26.18 | U7.2 20.9,34.55 21.72,35.37 v21.72,37.07 | C32.1 15.07,5.72 U9.2 | LED3.4 20.62,59.27 23.4,56.5 JP7.1 | J1.S3 J1.S4 J1.S5 | J1.S2 J1.5
  Top 0.305: C61.C 73.41,65.91 v75.69,65.91
  Top 0.406: v89.84,66.71 89.94,66.8 C76.C | C77.C 89.44,58.2 v88.75,57.51 87.35,58.91 IC5.1
  other vias: 47.15,42.41 48.65,42.41 51.65,42.41 53.15,42.41 54.65,42.41 47.15,41.01 48.65,41.01 50.15,41.01 51.65,41.01 53.15,41.01 54.65,41.01 47.15,39.61 48.65,39.61 50.15,39.61 51.65,39.61 53.15,39.61 54.65,39.61 47.15,38.11 48.65,38.11 50.15,38.11 51.65,38.11 53.15,38.11 54.65,38.11 47.15,36.61 48.65,36.61 50.15,36.61 51.65,36.61 53.15,36.61 54.65,36.61 47.15,35.21 48.65,35.21 50.15,35.21 51.65,35.21 53.15,35.21 54.65,35.21 37.65,20.9
  pour Bottom (isolate 0.012): 100.67,75.41 101,5.78 95.45,0.3 3.05,0.5 1.2,4.85 1.1,73.86 5.19,76.71 97.28,76.66
GPIO0  (via drill 0.5)
  Top 0.254: U2.42 41.4,36.8 40.95,36.35 34.3,36.35 26.15,28.2 26.15,14.55 v26.55,14.15
  Bottom 0.254: v26.55,14.15 26.55,13.55 32.9,7.2 32.9,4.3 34.02,3.18 U9.11
GPIO1  (via drill 0.5)
  Top 0.254: U2.43 42.25,36.3 41.75,35.8 35.95,35.8 34.3,34.15 33.25,34.15 26.95,27.85 26.95,16.35 v28,15.3
  Bottom 0.254: v28,15.3 34.17,9.13 U9.12
GPIO2
  Top 0.254: JP6.2 54.14,2.29 52.95,1.1 38.79,1.1 U9.13
GPIO3  (via drill 0.5)
  Top 0.254: JP6.3 56.68,6.37 55.85,7.2 49.55,7.2 v48,5.65
  Bottom 0.254: v48,5.65 45.4,8.25 39.24,8.25 U9.14
INTN  (via drill 0.5)
  Top 0.254: U2.45 37.75,35.3 35.3,32.85 33.15,32.85 27.7,27.4 27.7,18.5 v28.15,18.05 | v33.85,12.6 30.35,9.1 30.35,4.25 29.28,3.18 U9.7
  Bottom 0.254: v28.15,18.05 28.4,18.05 v33.85,12.6
MISO
  Top 0.254: U2.40 34.6,37.8 25.25,28.45 25.25,12.55 24.01,11.31 U9.4
MOSI  (via drill 0.5)
  Top 0.254: U2.39 34.15,38.3 23.6,27.75 v23.6,13.75
  Bottom 0.254: v23.6,13.75 25.25,12.1 25.25,4.15 26.22,3.18 U9.5
N$1
  Top 0.254: Y1.3 42.85,27.45 44.9,29.5 U2.51
N$2
  Top 0.254: R16.1 54.7,70.4 52.25,67.95 52.25,65.5 55.3,62.45 LED1.A
N$3
  Top 0.254: U2.50 41.6,32.8 39.65,30.85 Y1.1
N$4
  Top 0.254: L2.1 89.15,36.55 87.1,38.6 87.1,40 85.7,41.4 U4.15
N$5  (via drill 0.5)
  Top 0.254: U4.23 81.34,44.36 80.9,44.8 v80.5,44.8 | v82,37.3 81.3,36.6 SJ1.2
  Bottom 0.254: v80.5,44.8 79.6,43.9 79.6,40.3 82,37.9 v82,37.3
N$6
  Top 0.254: U4.1 79.5,43.51 R6.1 C6.1
N$7
  Top 0.254: L1.1 87.7,46.9 85.7,44.9 85.7,42.8 85.31,42.41 U4.17
N$8
  Top 0.254: J4.1 70.45,69.42 FB1.1
N$9
  Top 0.254: 70.54,67.73 70.58,67.7 C1.1
  Top 0.305: FB1.2 70.54,67.73 F1.1
N$10
  Top 0.254: U$2.1 11.43,69.17 11.78,68.82 SJ6.2
N$11
  Top 0.254: R14.1 66.5,70.2 62.92,66.62 U1.12
N$12
  Top 0.254: R15.1 62.8,68.7 U1.11
N$13
  Top 0.254: U4.10 82.35,38.25 84,36.6 84.1,36.6 84.4,36.3 SJ8.1
N$14
  Top 0.254: JP4.1 10.97,66.92 SJ6.3
N$15
  Top 0.254: R14.2 69.8,71.8 J4.2 69.8,73.8 70.2,74.2 73.5,74.2 73.7,74 C22.1
N$16
  Top 0.254: R15.2 65.8,71.5 68.7,71.5 69.15,71.95 J4.3 69.15,73.75 68.7,74.2 C23.1
N$17
  Top 0.254: X3.1 10.41,30.21 15.7,35.5 U7.4
N$18
  Top 0.254: R3.1 56.19,66.14 LED2.A
N$22
  Top 0.254: L1.2 94.65,48.25 93.95,48.95 90.9,48.95 90.4,48.45 89.09,48.45 SJ4.2 | L1.2 94.7,46.85 C8.1 R9.1 | C7.1 94.75,47 L1.2
N$24
  Top 0.254: Q3.1 73.66,60.5 R4.1
N$25
  Top 0.254: T1.3 58.72,56.67 C3.2 59.5,56.8 60,56.3 63.5,56.3 64.25,55.55 R1.3
N$28
  Top 0.254: U8.4 11.79,49.6 X2.1
N$29
  Top 0.254: U6.21 73.31,21.41 74.2,22.3 C73.1
N$30
  Top 0.254: C31.1 72.03,22.57 U6.24
N$31  (via drill 0.5 pad 0.3)
  Top 0.254: R17.1 62.8,14.9 v63.2,14.5 | v69.35,14.15 70.1,14.15 70.7,14.75 71.75,14.75 72.95,15.95 73.8,15.95 74.61,16.75 U6.13
  Bottom 0.254: v63.2,14.5 69,14.5 v69.35,14.15
N$32
  Top 0.254: SJ2.2 37.25,69.66 U$3.1
N$33
  Top 0.254: JP5.1 34.35,65.95 35.85,67.45 SJ2.3
N$34
  Top 0.254: C9.1 96.7,36.55 L2.2 | R7.1 C10.1 94.75,38.85 L2.2 | L2.2 94.9,36.4 SJ5.2
N$35  (via drill 0.5)
  other vias: 79.35,63.8
N$36  (via drill 0.5)
  other vias: 79.35,62.55
N$37  (via drill 0.5)
  other vias: 79.35,61.05
N$38  (via drill 0.5)
  other vias: 79.35,59.7
N$40
  Top 0.254: J1.2 8.75,63.4 9.5,62.65 9.5,61.7 JP8.1 10.4,60.8 10.4,59.95 9.25,58.8 SJ9.2
N$41
  Top 0.254: J1.3 5.91,62.75 JP8.2 6.8,60.04 SJ10.2
N$42
  Top 0.254: J1.1 6.86,64.05 SJ11.2
N$43
  Top 0.254: SJ3.2 83.9,27.05 85.1,25.85 91.1,25.85 93.55,23.4 96.8,23.4 97.77,24.37 U$1.2
N$45
  Top 0.254: LED5.A 71,55.37 R5.1
N$78
  Top 0.254: U10.3 20.68,15.27 21.95,14 21.95,10.45 20.9,9.4 19.2,9.4 17,11.6 C71.PPOS
N$79
  Top 0.254: U10.2 20.02,13.83 X5.P$1
N$81
  Top 0.254: X5.P$2 19.05,11.15 18.6,11.6 18.6,15.38 U10.1
P0
  Top 0.254: U2.3 55.9,49.65 57.5,51.25 57.5,58.75 50.8,65.45 50.8,73.05 U$3.10
P1
  Top 0.254: U2.4 55.4,50.05 56.9,51.55 56.9,58.3 49.53,65.67 U$3.9
P2
  Top 0.254: U$3.8 48.25,73.06 48.25,63.35 54.4,57.2 U2.6
P3
  Top 0.254: U2.7 53.9,56.9 46.99,63.81 U$3.7
P4
  Top 0.254: U2.9 52.9,56.75 45.75,63.9 45.75,73.02 U$3.6
P5
  Top 0.254: U2.10 52.4,56 44.45,63.95 U$3.5
P6
  Top 0.254: U2.12 51.4,54.7 43.2,62.9 43.2,73.15 42.03,74.32 U$3.4
P7
  Top 0.254: U2.13 50.9,53.75 41.91,62.74 U$3.3
P8
  Top 0.254: U$2.10 22.85,72.91 22.85,69.85 36.15,56.55 45.55,56.55 49.9,52.2 U2.15
P9
  Top 0.254: U2.16 49.4,52 45.4,56 35.25,56 21.59,69.66 U$2.9
P10
  Top 0.254: U$2.8 20.3,72.92 20.3,70 34.95,55.35 42.55,55.35 48.4,49.5 U2.18
P11
  Top 0.254: U2.19 47.9,49.3 42.5,54.7 34.55,54.7 19.05,70.2 U$2.7
P12
  Top 0.254: U$2.6 17.8,72.88 17.8,70.35 34.15,54 42.45,54 46.9,49.55 U2.21
P13
  Top 0.254: U2.22 46.4,49.1 42.1,53.4 33.65,53.4 16.51,70.54 U$2.5
P14
  Top 0.254: U$2.4 15.25,72.89 15.25,70.3 32.95,52.6 38.85,52.6 43.4,48.05 45,48.05 45.4,47.65 U2.24
P15
  Top 0.254: U2.25 43.78,46.47 38.3,51.95 32.45,51.95 13.97,70.43 U$2.3
P16
  Top 0.254: U2.27 42.1,44.3 40.95,45.45 33.7,45.45 27.44,51.71 JP7.2 20.14,51.71 17.8,54.05 17.8,58.8 17.35,59.25 15.97,59.25 LED3.1
P32
  Top 0.152: 47.89,16.62 47.39,17.12 47.4,21.05 47.14,21.29 47.14,22.46
  Top 0.254: U5.P$18 47.89,16.62 | U2.53 45.9,28 44.8,26.9 44.8,24.9 47.14,22.46
P33  (via drill 0.3 pad 0.3, 0.5)
  Top 0.152: U5.P$17 47.39,15.02 47.39,13.92 47.59,13.72 47.59,13.22 47.29,12.92
  Top 0.254: v42.19,17.82 42.79,17.82 44.6,19.63 v44.6,23.1 | v42.49,14.22 43.95,12.75 47.12,12.75 47.29,12.92 | U2.54 46.4,26.7 v45.6,25.9
  Bottom 0.254: v42.19,17.82 42.49,17.52 v42.49,14.22 | v45.6,25.9 45.6,24.1 v44.6,23.1
P34  (via drill 0.5)
  Top 0.152: U5.P$14 46.39,18.02 46.39,20.22
  Top 0.254: U2.56 47.4,27.8 48.1,27.1 48.1,24.3 v47.4,23.6 | v46,22.2 46,20.6 46.39,20.22
  Bottom 0.254: v47.4,23.6 v46,22.2
P35
  Top 0.152: U5.P$19 48.39,18.02 48.39,20.82
  Top 0.254: 48.39,20.82 49.19,21.62 49.19,22.61 48.8,23 48.8,27.2 48.5,27.5 48.5,27.6 47.9,28.2 U2.57
P36  (via drill 0.5)
  Top 0.152: U5.P$20 47.89,20.92
  Top 0.254: U2.59 48.9,29.2 v48.65,28.9 | v48.1,21.9 47.89,21.69 47.89,20.92
  Bottom 0.254: v48.65,28.9 48.6,22.4 v48.1,21.9
P37
  Top 0.152: 50.39,17.92 48.99,16.52
  Top 0.254: U5.P$23 48.99,16.52 | 50.39,17.92 50.39,19.02 51.49,20.12 51.49,21.01 50.8,21.7 50.1,21.7 49.7,22.1 49.7,23 49.4,23.3 U2.60
P38
  Top 0.152: 48.79,15.52 48.39,15.12 48.39,14.12 48.79,13.72
  Top 0.254: 48.79,15.52 U5.P$22 50.25,15.52 52.2,17.46 52.2,22.2 50.4,24 U2.62 | 48.79,13.72 49.89,13.72
P39
  Top 0.152: U5.P$21 49.89,14.52
  Top 0.254: U2.63 50.9,24.5 52.9,22.5 52.9,16.9 50.52,14.52 49.89,14.52
P40  (via drill 0.3 pad 0.3, 0.5)
  Top 0.152: U5.P$7 44.39,14.02
  Top 0.254: 44.39,14.02 44.39,13.52 v44.29,13.52 | U2.65 51.9,24.6 53.8,22.7 53.8,14.5 51.1,11.8 44.5,11.8 v44.4,11.9
  Bottom 0.254: v44.4,11.9 44.39,11.91 44.39,13.42 v44.29,13.52
P41  (via drill 0.5)
  Top 0.152: U5.P$13 47.39,16.02 49.59,16.02
  Top 0.254: U2.66 52.4,24.9 54.8,22.5 54.8,19.9 v55.2,19.5 | v51.3,18.3 51.3,17.73 49.59,16.02
  Bottom 0.254: v55.2,19.5 52.5,19.5 v51.3,18.3
P42
  Top 0.152: U5.P$3 43.49,16.52
  Top 0.254: 43.49,16.52 41.79,14.82 41.79,13.72 43.19,12.42 43.2,12.4 43.2,11.4 44,10.6 51.2,10.6 54.9,14.3 54.9,17 56.5,18.6 56.5,19.9 55.9,20.5 55.9,23.9 53.4,26.4 U2.68
P43
  Top 0.152: U5.P$4 43.49,17.52
  Top 0.254: 43.49,17.52 41.09,15.12 41.09,12.11 43.3,9.9 51.6,9.9 56.3,14.6 56.3,15.5 57.1,16.3 57.1,23.6 53.9,26.8 U2.69
P48
  Top 0.254: U2.77 61.8,33.3 63.9,31.2 69.4,31.2 80.8,19.8 88.3,19.8 92.5,15.6 92.5,14.3 93.6,13.2 96.35,13.2 97.64,14.49 U$1.10
P49
  Top 0.254: U2.78 62.1,33.8 64,31.9 69.7,31.9 81.2,20.4 88.7,20.4 94.61,14.49 U$1.9
P50
  Top 0.254: U2.80 67.9,34.8 81.5,21.2 88.8,21.2 94.25,15.75 96.45,15.75 97.73,17.03 U$1.8
P51
  Top 0.254: U2.81 68.6,35.3 81.9,22 88.9,22 93.87,17.03 U$1.7
P52
  Top 0.254: U2.83 59.5,36.3 60,35.8 69.5,35.8 82.7,22.6 89.2,22.6 93.5,18.3 96.3,18.3 97.57,19.57 U$1.6
P53
  Top 0.254: U2.84 59.8,36.8 60.3,36.3 70.1,36.3 83.1,23.3 89.5,23.3 93.23,19.57 U$1.5
P54
  Top 0.254: U2.86 61.2,37.8 62.1,36.9 70.8,36.9 83.8,23.9 89.8,23.9 92.85,20.85 96.3,20.85 97.56,22.11 U$1.4
P55
  Top 0.254: U2.87 61.5,38.3 62.2,37.6 71.1,37.6 84.3,24.4 90.5,24.4 92.79,22.11 U$1.3
PDN
  Top 0.254: U2.49 40.9,33.3 36.4,28.8 33.5,28.8 31.95,27.25 31.95,13.7 29.09,10.84 U9.8
PWREN  (via drill 0.5)
  Top 0.254: U1.19 64.08,62.08 v64.25,61.9 | v74.35,58 75.1,58 R4.2 76.6,58.7 76.9,59 76.9,61.3 76.1,62.1 R18.1
  Bottom 0.254: v74.35,58 72.3,60.05 69.4,60.05 67.55,61.9 v64.25,61.9
RST  (via drill 0.5)
  Top 0.254: 60.76,50.7 T1.1 61.51,54.83 R1.4 | 60.76,50.7 60.76,48.51 60.1,47.85 60.1,46.33 U2.100 | SJ8.2 84.4,33 | 84.4,33 84.4,32.5 82.8,30.9 78.8,30.9 73.6,36.1 73.6,37.7 71.4,39.9 68.4,39.9 v67.9,40.4 | v62.3,50.7 60.76,50.7 | S2.2 86,33 84.4,33
  Top 0.406: S2.3 S2.2
  Bottom 0.254: v67.9,40.4 67.9,49.4 66.8,50.5 62.5,50.5 v62.3,50.7
RX
  Top 0.254: U2.98 60.4,43.8 61.55,44.95 61.55,46.7 67.3,52.45 67.3,56.1 65.65,57.75 65.65,62.9 66.12,63.38 U1.4
RXLED
  Top 0.254: U1.17 60.02,63.38 58.91,64.5 LED2.C
SCK
  Top 0.254: U2.46 38.35,34.8 35.05,31.5 32.85,31.5 29.35,28 29.35,14.75 25.25,10.65 25.25,3.95 24.48,3.18 U9.3
SCL  (via drill 0.3 pad 0.3, 0.5 pad 0.3)
  Top 0.254: U2.89 59.8,39.3 v60.1,39.55 | v67.7,30.4 67.7,28.4 70.3,25.8 70.3,21.95 | 70.3,21.95 70.3,20.45 70.95,19.8 U6.2 | R17.3 62.1,16.5 62.45,16.85 62.45,20.75 v62.6,20.9 | v69.2,21.95 70.3,21.95
  Bottom 0.254: v60.1,39.55 58.6,38.15 58.6,35.3 61.8,32.1 66,32.1 v67.7,30.4 | v62.6,20.9 66.65,20.9 67.6,21.85 69.1,21.85 v69.2,21.95
SCL_N1
  Top 0.254: U2.37 34.2,39.3 33.05,40.45 31.1,40.45 25.5,34.85 25.5,31.6 22.85,28.95 22.85,19.85 21.85,18.85 21.15,18.85 20.68,19.32 U10.6
SD_CLK
  Top 0.254: U2.72 55.4,29.1 57.5,27 59.2,27 65.8,20.4 65.8,14.1 73.2,6.7 76.1,6.7 77.55,5.25 U$35.CLK
SD_CS
  Top 0.254: U2.75 57.67,31.13 60,28.8 63.2,28.8 64.8,27.2 65.5,27.2 67.2,25.5 67.2,14.6 73.6,8.2 78.2,8.2 80.85,5.55 U$35.CD/DAT3
SD_MISO
  Top 0.254: U2.71 54.9,28.6 57.2,26.3 58.9,26.3 64.5,20.7 64.5,14.5 70.6,8.4 70.6,7.5 72,6.1 74.5,6.1 75.35,5.25 U$35.DAT0
SD_MOSI
  Top 0.254: U2.74 56.4,30.1 56.9,29.6 58.1,29.6 59.5,28.2 62.3,28.2 64.2,26.3 65.5,26.3 66.5,25.3 66.5,14.4 73.4,7.5 77.6,7.5 79.75,5.35 U$35.CMD
SDA  (via drill 0.3 pad 0.3, 0.5 pad 0.3)
  Top 0.254: U2.90 57.3,39.8 v56.9,40.2 | v65.7,30.3 65.7,28.9 67.95,26.6 67.95,21.5 68.33,21.12 | 68.33,21.12 70.52,18.93 U6.4 | R17.2 62.8,15.7 63.2,16.1 63.2,19.15 v63.5,19.45 | v68.15,19.95 68.15,20.95 68.33,21.12
  Bottom 0.254: v56.9,40.2 56.9,35.2 60.9,31.2 64.8,31.2 v65.7,30.3 | v63.5,19.45 67.65,19.45 v68.15,19.95
SDA_N1
  Top 0.254: U2.36 36.55,39.8 35.25,41.1 30.85,41.1 24.95,35.2 24.95,32.1 22.35,29.45 22.35,21.47 U10.5
TO5V  (via drill 0.5)
  Top 0.254: SJ7.1 82.55,53.9 82.25,53.6 80.95,53.6 79.45,52.1 v79.45,49.2 79.45,47.75 R6.2 83.3,47.7 C5.1 | U4.20 82.86,44.61 83.4,45.15 C5.1 | U4.2 79.29,42.41 v78,43.7 | U4.8 81.34,38.94 v80.25,37.85 80.49,37.61 SJ1.3 80.49,34.46 82.15,32.8 v82.15,31.7 | U4.16 86.75,41.9 v87.8,42.95 | v85.1,47.7 85,47.8 C5.1 | v84.2,30.85 83.9,30.55 SJ3.1
  Bottom 0.254: v79.45,49.2 78,47.75 v78,43.7 78,40.1 v80.25,37.85 | v87.8,42.95 88.55,43.7 88.55,46.6 87.45,47.7 v85.1,47.7 | v82.15,31.7 83,30.85 v84.2,30.85
TX
  Top 0.254: U2.99 59.8,44.3 60.85,45.35 60.85,46.95 66.75,52.85 66.75,55.8 64.6,57.95 64.6,59.9 64.1,60.4 62.3,60.4 61.38,61.33 U1.20
TXLED
  Top 0.254: U1.18 59.83,62.73 59.55,62.45 LED1.C
USB_ENABLE  (via drill 0.5)
  Top 0.254: U2.28 41.7,43.8 40.9,44.6 26.95,44.6 25.82,43.48 | 25.82,43.48 24.2,41.85 21.4,41.85 21.1,42.15 U8.1 | U7.1 21.55,33.6 v21.7,33.75 | v21.55,45.4 23.9,45.4 25.82,43.48
  Bottom 0.254: v21.7,33.75 21.7,34.8 20.15,36.35 20.15,44 v21.55,45.4
VLDO1
  Top 0.254: U4.3 77,41.9 R13.1 76.9,42.2 C12.1 74.05,43.2 JP2.1
VLDO2
  Top 0.254: R11.1 77.5,36.8 | 77.5,36.8 80.37,39.67 U4.7 | 77.5,36.8 78.1,36.2 C13.1 78.9,35.4 79.2,35.1 79.2,34.7 79.35,34.55 79.35,33.45 JP3.1
WALL_POWER
  Top 0.406: J6.1 87.35,66.75 IC5.3 87.39,64 C76.A
(copper drawn outside any net)
  shapes: Bottom area x1, Top area x1

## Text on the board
tPlace: USB | GND | P16 | +3.3 | P2 Board1 Rev.4B | Audio | GPIO2 | GPIO3 | GND | 3.3V | 5V | 1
